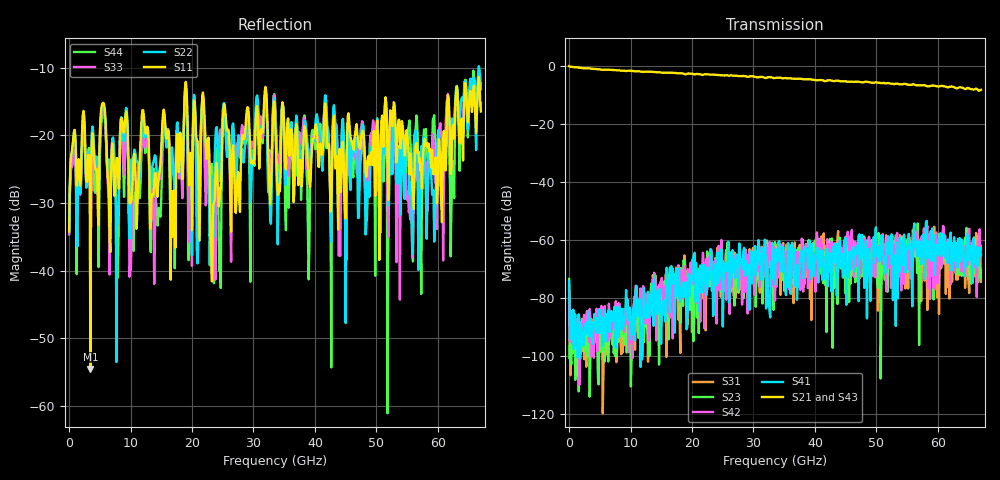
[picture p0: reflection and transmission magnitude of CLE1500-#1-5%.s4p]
!Keysight Technologies,N5247B,US50470101,A.16.20.02
!Date: Thursday, March 13, 2025 10:09:27
!Correction: S11(C  4-Port  )
!S12(C  4-Port  )
!S13(C  4-Port  )
!S14(C  4-Port  )
!S21(C  4-Port  )
!S22(C  4-Port  )
!S23(C  4-Port  )
!S24(C  4-Port  )
!S31(C  4-Port  )
!S32(C  4-Port  )
!S33(C  4-Port  )
!S34(C  4-Port  )
!S41(C  4-Port  )
!S42(C  4-Port  )
!S43(C  4-Port  )
!S44(C  4-Port  )
!S4P File: Measurements: <S11,S12,S13,S14>,
!<S21,S22,S23,S24>,
!<S31,S32,S33,S34>,
!<S41,S42,S43,S44>:
# Hz S  dB  R 50
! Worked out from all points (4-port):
!   601 points, 10 MHz to 67 GHz, reference 50 ohm
!   strongest paths, dB at 10 MHz, 16.76 GHz, 33.51 GHz, 50.25 GHz, 67 GHz:
!     S21: 0.0, -2.3, -4.1, -5.7, -8.2
!     S43: 0.0, -2.4, -4.3, -5.6, -8.3
!     S41: -74.3, -74.8, -75.4, -63.7, -65.4
!     S42: -77.8, -75.4, -81.0, -67.4, -63.3
!     S23: -73.5, -75.3, -60.8, -76.5, -73.0
!     S31: -75.9, -85.4, -62.5, -84.5, -74.5
!   lowest |S11| = -54.5 dB at 3.471 GHz (marker M1), VSWR 1.00, Z = 50 + j0.187 ohm
!   |S11| at or under -10 dB: start of sweep to end of sweep
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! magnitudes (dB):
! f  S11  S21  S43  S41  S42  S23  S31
! 10 MHz  -34.2  0.0  0.0  -74.3  -77.8  -73.5  -75.9
! 3.471 GHz  -54.5  -0.8  -0.8  -87.4  -86.9  -101.0  -92.0
! 5.481 GHz  -15.2  -1.3  -1.2  -96.7  -95.5  -97.4  -119.9
! 7.825 GHz  -23.3  -1.4  -1.4  -87.5  -84.1  -94.9  -97.6
! 18.99 GHz  -12.1  -2.8  -2.8  -74.6  -73.3  -74.2  -72.7
! 57.17 GHz  -25.3  -6.7  -7.2  -65.2  -59.9  -67.3  -60.6
! 67 GHz  -16.5  -8.2  -8.3  -65.4  -63.3  -73.0  -74.5
